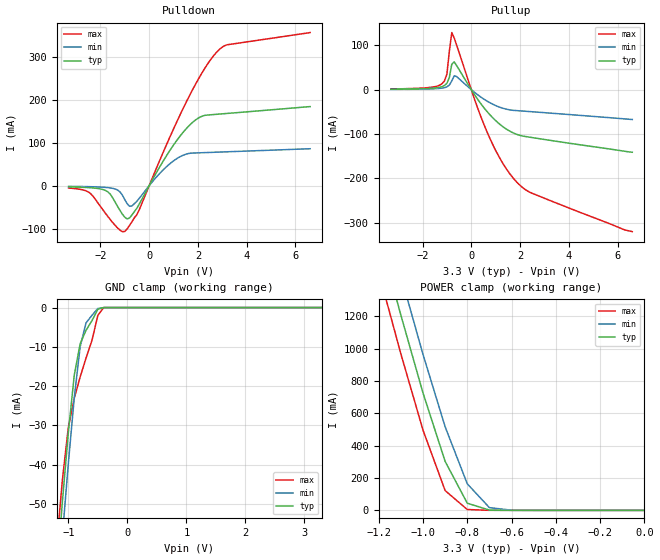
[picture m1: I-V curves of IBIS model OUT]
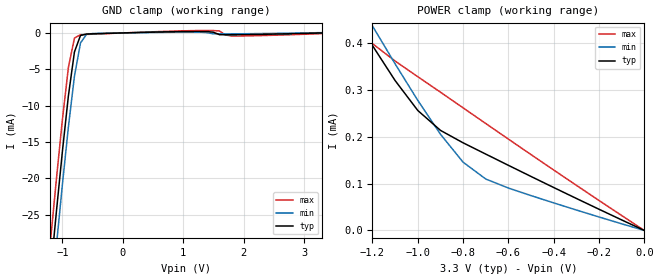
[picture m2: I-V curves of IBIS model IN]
|   TEXAS INSTRUMENTS INCORPORATED
|   Standard Linear and Logic
|   IBIS Model of ALVCH16820
|   10-Bit Flip-Flop With Dual Outputs and 3-State Outputs
|   TSSOP 56-pin (DGG) Package
[IBIS Ver]   2.1
[Comment char]  |_char
[File Name]   alh16820.ibs
[File Rev]   2.0
[Date]   8/11/98
[Source]   File originated at Texas Instruments, Inc.
[Notes]   The following is an IBIS list for the ALVCH16820.
|   - All test data contained in this file are derived from
|   hspice(tm) simulations.
|   - File created by David Yaeger, SLL Applications
|   - This file may be incomplete or may not be fully compliant
|   with the IBIS specification. It will be replaced with a
|   version that is IBIS Revision 3.2 compliant and is complete
|   and accurate.
|   Please email all questions and comments to sllibis@ti.com.
[Disclaimer]
* Property of Texas Instruments Incorporated.  Unauthorized *
* reproduction and/or distribution is strictly prohibited. *
* This product is protected under copyright law. *
* Created 1997, (C) Copyright 1997, Texas Instruments Inc., *
* All Rights Reserved *
* UNLESS THERE IS A SIGNED, WRITTEN AGREEMENT TO THE *
* CONTRARY, TEXAS INSTRUMENTS ("TI") IS PROVIDING THE IBIS *
* MODELS "AS IS" AND WITHOUT ANY WARRANTY, EXPRESSED OR *
* IMPLIED.  TI assumes no liability for: *
* 1) the accuracy of the IBIS models provided to your *
* company; *
* 2) the proper functioning of these IBIS models in your *
* design or for any resulting applications; or *
* 3) infringement of patents, copyrights or intellectual *
* property rights resulting from your use of these *
* IBIS models. *
* TI provides IBIS Models as a service to our customers. *
* You and your company shall not distribute, sell or give *
* these models to anyone else without prior written *
* permission from TI. *
* TI reserves the right to make changes to our products or *
* to discontinue any semiconductor product or service *
* without notice, and advises our customers to obtain the *
* latest version of relevant information to verify, before *
* placing orders, that the information being relied on is *
* current. *
* Please be aware that your receipt and use of the IBIS *
* information provided shall serve as acceptance of these *
* terms and conditions.  If you do not accept these terms,	  *
* you should return or destroy the IBIS models and any *
* other accompanying information immediately. *
[Component]   ALVCH16820_DGG
[Manufacturer]  Texas Instruments, Inc.
[Package]
|   typ   min   max
R_pkg   0.022   0.020   0.025
L_pkg   3.48nH   1.75nH   5.20nH
C_pkg   0.33pF   0.16pF   0.49pF
[Pin]   signal_name   model_name   R_pin   L_pin   C_pin
1   1OE   NC   0.062   5.094nH   0.856pF
2   1Q1   OUT   0.061   4.621nH   0.902pF
3   1Q2   OUT   0.060   4.316nH   0.802pF
4   GND   GND   0.059   3.968nH   0.698pF
5   2Q1   OUT   0.057   3.716nH   0.649pF
6   2Q2   OUT   0.042   3.517nH   0.652pF
7   VCC   POWER   0.041   3.160nH   0.570pF
8   3Q1   OUT   0.039   2.981nH   0.482pF
9   3Q2   OUT   0.039   2.809nH   0.447pF
10   4Q1   OUT   0.038   2.715nH   0.409pF
11   GND   GND   0.041   2.675nH   0.391pF
12   4Q2   OUT   0.039   2.536nH   0.366pF
13   5Q1   OUT   0.039   2.457nH   0.348pF
14   5Q2   OUT   0.038   2.411nH   0.353pF
15   6Q1   OUT   0.039   2.456nH   0.355pF
16   6Q2   OUT   0.039   2.471nH   0.349pF
17   7Q1   OUT   0.040   2.580nH   0.370pF
18   GND   GND   0.038   2.651nH   0.389pF
19   7Q2   OUT   0.038   2.739nH   0.411pF
20   8Q1   OUT   0.038   2.739nH   0.411pF
21   8Q2   OUT   0.038   2.988nH   0.484pF
22   VCC   POWER   0.038   3.105nH   0.564pF
23   9Q1   OUT   0.040   3.427nH   0.638pF
24   9Q2   OUT   0.056   3.654nH   0.641pF
25   GND   GND   0.057   3.932nH   0.700pF
26   10Q1   OUT   0.058   4.257nH   0.806pF
27   10Q2   OUT   0.057   4.580nH   0.914pF
28   2OE   NC   0.059   5.038nH   0.861pF
29   NC   NC   0.060   5.058nH   0.858pF
30   NC   NC   0.056   4.543nH   0.904pF
31   D10   IN   0.057   4.240nH   0.803pF
32   GND   GND   0.057   3.929nH   0.700pF
33   NC   NC   0.056   3.616nH   0.637pF
34   D9   IN   0.037   3.368nH   0.640pF
35   VCC   POWER   0.036   3.024nH   0.563pF
36   NC   NC   0.035   2.876nH   0.474pF
37   D8   IN   0.035   2.745nH   0.444pF
38   NC   NC   0.037   2.683nH   0.405pF
39   GND   GND   0.038   2.603nH   0.382pF
40   D7   IN   0.038   2.510nH   0.362pF
41   NC   NC   0.036   2.412nH   0.341pF
42   D6   IN   0.038   2.416nH   0.349pF
43   NC   NC   0.037   2.403nH   0.349pF
44   D5   IN   0.037   2.429nH   0.341pF
45   NC   NC   0.036   2.482nH   0.358pF
46   GND   GND   0.037   2.615nH   0.381pF
47   D4   IN   0.035   2.669nH   0.402pF
48   NC   NC   0.036   2.763nH   0.442pF
49   D3   IN   0.036   2.942nH   0.478pF
50   VCC   POWER   0.035   3.053nH   0.564pF
51   NC   NC   0.036   3.409nH   0.641pF
52   D2   IN   0.058   3.698nH   0.641pF
53   GND   GND   0.059   3.975nH   0.697pF
54   NC   NC   0.061   4.327nH   0.802pF
55   D1   IN   0.061   4.624nH   0.905pF
56   CLK   NC   0.060   5.063nH   0.858pF
|   Component ALVCH16820_DL
[Component]   ALVCH16820_DL
[Manufacturer]  Texas Instruments, Inc.
[Package]
|   typ   min	max
R_pkg   0.055   0.048	0.067
L_pkg   6.539nH   4.802nH	9.746nH
C_pkg   0.857pF   0.5pF	1.351pF
[Pin]	signal_name	  model_name   R_pin	 L_pin	C_pin
1	1OE   NC   0.064	9.646nH	1.202pF
2	1Q1   OUT   0.059	8.723nH	1.348pF
3	1Q2   OUT   0.059	8.139nH	1.223pF
4	GND   GND   0.056	7.554nH	1.088pF
5	2Q1   OUT   0.054	6.991nH	0.966pF
6	2Q2   OUT   0.053	6.659nH	0.973pF
7	VCC   POWER   0.055	6.321nH	0.905pF
8	3Q1   OUT   0.055	5.942nH	0.713pF
9	3Q2   OUT   0.057	5.767nH	0.678pF
10	4Q1   OUT   0.054	5.459nH	0.631pF
11	GND   GND   0.051	5.224nH	0.638pF
12	4Q2   OUT   0.048	5.088nH	0.601pF
13	5Q1   OUT   0.05	5.021nH	0.518pF
14	5Q2   OUT   0.051	4.802nH	0.5pF
15	6Q1   OUT   0.051	4.803nH	0.5pF
16	6Q2   OUT   0.05	5.021nH	0.518pF
17	7Q1   OUT   0.048	5.088nH	0.601pF
18	GND   GND   0.051	5.224nH	0.638pF
19	7Q2   OUT   0.054	5.459nH	0.631pF
20	8Q1   OUT   0.057	5.768nH	0.677pF
21	8Q2   OUT   0.055	5.942nH	0.715pF
22	VCC   POWER   0.055	6.321nH	0.907pF
23	9Q1   OUT   0.053	6.659nH	0.972pF
24	9Q2   OUT   0.054	6.991nH	0.966pF
25	GND   GND   0.056	7.554nH	1.087pF
26	10Q1   OUT   0.059	8.139nH	1.223pF
27	10Q2   OUT   0.059	8.727nH	1.351pF
28	2OE   NC   0.067	9.746nH	1.21pF
29	NC   NC   0.063	9.63nH	1.203pF
30	NC   NC   0.06	8.751nH	1.349pF
31	D10   IN   0.06	8.184nH	1.224pF
32	GND   GND   0.056	7.543nH	1.087pF
33	NC   NC   0.054	7.005nH	0.969pF
34	D9   IN   0.056	6.714nH	0.975pF
35	VCC   POWER   0.058	6.384nH	0.909pF
36	NC   NC   0.057	5.976nH	0.717pF
37	D8   IN   0.057	5.743nH	0.677pF
38	NC   NC   0.055	5.469nH	0.631pF
39	GND   GND   0.055	5.328nH	0.644pF
40	D7   IN   0.052	5.189nH	0.606pF
41	NC   NC   0.052	5.053nH	0.519pF
42	D6   IN   0.052	4.825nH	0.502pF
43	NC   NC   0.054	4.896nH	0.506pF
44	D5   IN   0.052	5.093nH	0.521pF
45	NC   NC   0.051	5.179nH	0.608pF
46	GND   GND   0.054	5.314nH	0.645pF
47	D4   IN   0.055	5.511nH	0.632pF
48	NC   NC   0.057	5.77nH	0.677pF
49	D3   IN   0.055	5.956nH	0.716pF
50	VCC   POWER   0.055	6.32nH	0.905pF
51	NC   NC   0.052	6.621nH	0.968pF
52	D2   IN   0.053	6.974nH	0.966pF
53	GND   GND   0.057	7.571nH	1.089pF
54	NC   NC   0.057	8.097nH	1.219pF
55	D1   IN   0.059	8.723nH	1.349pF
56	CLK   NC   0.061	9.56nH	1.199pF
| Models and submodels in the file (2): OUT (3-state), IN (Input)
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|   Model ALVCH16820_OUT
[Model]   OUT
Model_type   3-state
Polarity   Non-Inverting
Enable   Active-Low
|Variable   typ   min   max
C_comp   7.0pF   NA   NA
[Voltage range]   3.3   3.0   3.6
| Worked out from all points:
|   slope of the pulldown table from 0 to 0.495 V, typ, clamps not added: 9.96 ohm
|   slope of the pullup table from 0 to 0.495 V, typ, clamps not added: 12.6 ohm
|   GND clamp passes 1 mA (typ) near -0.52 V on its own axis
|   POWER clamp passes 1 mA (typ) near -0.66 V on its own axis
[Pullup]   | Note: Vtable = Vcc - Voutput
|   Voltage   I(typ)   I(min)   I(max)
-3.3V     1mA        600uA      1.7mA
-1.2V     6.7mA      3.4mA      13.3mA
-1V       14.29mA    6.322mA    35.01mA
-900mV    27.23mA    10.23mA    86.35mA
-800mV    57.41mA    19.92mA    128.7mA
-700mV    62.45mA    31.18mA    116.2mA
-600mV    54.15mA    29.3mA     100.1mA
600mV     -46.39mA   -24.34mA   -89.47mA
1.2V      -79.51mA   -40.29mA   -157.5mA
1.8V      -99.5mA    -47.06mA   -204.7mA
2.5V      -108.1mA   -49.91mA   -233.8mA
6.6V      -141.2mA   -67.38mA   -320.2mA
[Pulldown]
|   Voltage   I(typ)   I(min)   I(max)
-3.3V     -2.408mA   -1.238mA   -5.173mA
-2.5V     -4.052mA   -1.9mA     -13.88mA
-1.8V     -10.45mA   -3.578mA   -62.91mA
-1.3V     -46.98mA   -9.48mA    -97.3mA
-1V       -72.62mA   -31.54mA   -106.1mA
-700mV    -67.42mA   -46.46mA   -83.03mA
600mV     59.55mA    38.35mA    80.77mA
1.5V      131.2mA    73.24mA    191.8mA
2.1V      159.8mA    76.72mA    255.7mA
2.8V      166.2mA    78.17mA    312.1mA
3.2V      168mA      79.01mA    327.4mA
6.6V      183.9mA    86.1mA     355.8mA
[POWER_Clamp]   | Note: Vtable = Vcc - Voutput
|   Voltage   I(typ)   I(min)   I(max)
-3.3V     13.15A     13.37A     12.95A
-1.2V     1.712A     1.957A     1.472A
-1.1V     1.207A     1.45A      967.4mA
-1V       726mA      964.2mA    495.9mA
-900mV    302.7mA    516.7mA    122.4mA
-800mV    44.2mA     164mA      5.222mA
-700mV    1.634mA    16.95mA    93.3uA
-600mV    43.98uA    914.4uA    883.4nA
0V        660pA      601.1pA    720pA
[GND_Clamp]
|   Voltage   I(typ)   I(min)   I(max)
-3.3V     -499.7mA   -508.2mA   -491.7mA
-1.2V     -68.11mA   -77.06mA   -60.99mA
-1.1V     -49.34mA   -58.01mA   -43.79mA
-1V       -31.82mA   -39.74mA   -30.52mA
-900mV    -17.27mA   -23.03mA   -23.1mA
-800mV    -9.221mA   -9.981mA   -17.7mA
-700mV    -5.789mA   -3.91mA    -12.85mA
-600mV    -3.341mA   -1.966mA   -8.389mA
-500mV    -424.2uA   -244.6uA   -1.974mA
-400mV    -2.731nA   -92.41nA   -890.3pA
3.3V      660pA      72.23nA    600pA
[Ramp]
| variable   typ   min   max
dV/dt_r   1.5711E+00/1.7149E-10  1.1619E+00/2.5370E-10  1.9225E+00/1.5861E-10
dV/dt_f   1.6561E+00/1.1364E-10  1.3846E+00/2.6582E-10  1.8891E+00/9.6520E-11
|   Model ALVCH16820_IN
[Model]   IN
Model_type   Input
Polarity   Non-Inverting
Vinl = 0.8V
Vinh = 2.0V
|Variable   typ   min   max
C_comp   6pF   NA   NA
[Voltage Range]   3.3   3.0   3.6
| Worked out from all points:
|   GND clamp passes 1 mA (typ) near -0.73 V on its own axis
|   POWER clamp passes 1 mA (typ) near -1.92 V on its own axis
[POWER_Clamp]   | Note: Vtable = Vcc - Voutput
|   Voltage   I(typ)   I(min)   I(max)
-3.3V     2.214mA    2.263mA    2.166mA
-1.3V     474.5uA    519.7uA    452.7uA
-1.2V     394.9uA    436.8uA    399uA
-1.1V     320.2uA    355.8uA    361.8uA
-1V       256.3uA    277.8uA    328.4uA
-900mV    213.8uA    205.6uA    295.4uA
-800mV    187.2uA    145.8uA    261.9uA
-700mV    163.1uA    109.9uA    228.4uA
-600mV    139.1uA    90.61uA    195.1uA
-500mV    115.3uA    74.47uA    162uA
0V        1.111nA    1.078nA    1.126nA
[GND_Clamp]
|   Voltage   I(typ)   I(min)   I(max)
-3.3V     -229mA     -233.2mA   -224.9mA
-1.2V     -33.38mA   -38.07mA   -28.89mA
-1.1V     -24.69mA   -29.35mA   -20.22mA
-1V       -16.33mA   -20.9mA    -11.97mA
-900mV    -8.634mA   -12.92mA   -4.731mA
-800mV    -2.611mA   -5.945mA   -704.5uA
-700mV    -351.1uA   -1.372mA   -247.4uA
-600mV    -152.2uA   -189.2uA   -203.7uA
-500mV    -120.9uA   -82.4uA    -169uA
1.4V      187.2uA    34.98uA    335.9uA
1.8V      -248.2uA   -126.4uA   -424.2uA
3.3V      1.109nA    43.67uA    -93.16uA
